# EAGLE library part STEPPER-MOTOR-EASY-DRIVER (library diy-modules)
Stepper Motor Easy Driver Project page: http://www.schmalzhaus.com/EasyDriver/ Click here to find device on ebay.com
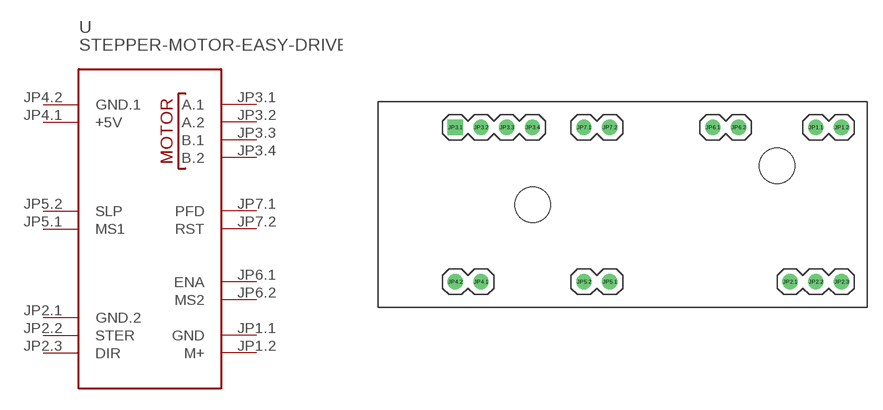
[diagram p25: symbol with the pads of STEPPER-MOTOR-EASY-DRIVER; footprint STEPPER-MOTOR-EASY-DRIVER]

Designator prefix -

## STEPPER-MOTOR-EASY-DRIVER  [STEPPER-MOTOR-EASY-DRIVER]
JP1.1  GND
JP1.2  M+
JP2.1  GND.2
JP2.2  STER
JP2.3  DIR
JP3.1  A.1
JP3.2  A.2
JP3.3  B.1
JP3.4  B.2
JP4.1  +5V
JP4.2  GND.1
JP5.1  MS1
JP5.2  SLP
JP6.1  ENA
JP6.2  MS2
JP7.1  PFD
JP7.2  RST

## Footprint STEPPER-MOTOR-EASY-DRIVER (pad centres in mm)
Stepper Motor Easy Driver
drill 1: JP1.1 19.05,7.62; JP1.2 21.59,7.62; JP2.1 16.51,-7.62; JP2.2 19.05,-7.62; JP2.3 21.59,-7.62; JP3.2 -13.97,7.62; JP3.3 -11.43,7.62; JP3.4 -8.89,7.62; JP4.1 -13.97,-7.62; JP4.2 -16.51,-7.62; JP5.1 -1.27,-7.62; JP5.2 -3.81,-7.62; JP6.1 8.89,7.62; JP6.2 11.43,7.62; JP7.1 -3.81,7.62; JP7.2 -1.27,7.62
drill 1 square: JP3.1 -16.51,7.62
hole 3.5 at -8.89,0
hole 3.5 at 15.24,3.81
